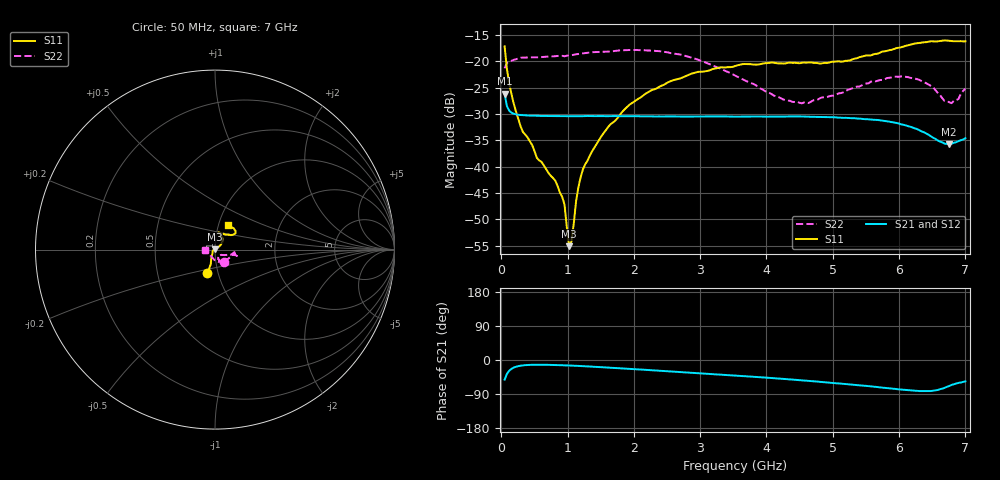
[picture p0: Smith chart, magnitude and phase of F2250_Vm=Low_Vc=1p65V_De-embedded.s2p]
! Integrated Device Technology
! Corporate Headquarters
! 6024 Silver Creek Valley Road
! San Jose, CA 95138  USA
! Phone:  1-408-284-8200
! Toll Free:  1-800-223-1366
! Webpage:  http://www.idt.com/
! Timing and RF Division
! 515 Groton Road, Suite 102
! Westford, MA 01886-6024
! Device:  F2250
! Description: Voltage Variable RF Attenuator
! Frequency:  50.0 -  6000.00 MHz
! Package:  3x3 mm Thin QFN Plastic Package: 16 pin
! Ports:  2 RF, 3 DC
!  Pin  1  = GND
!  Pin  2  = NC
!  Pin  3  = RF1  = Port 1
!  Pin  4  = NC
!  Pin  5  = GND
!  Pin  6  = GND
!  Pin  7  = GND
!  Pin  8  = GND
!  Pin  9  = NC
!  Pin 10  = RF2  = Port 2
!  Pin 11  = NC
!  Pin 12  = GND
!  Pin 13  = GND
!  Pin 14  = VCNTRL
!  Pin 15  = VDD
!  Pin 16  = VMODE
! Vcntrl:  1.650 Volts
! Vmode:  +0.000 Volts
! Vdd:  +3.30  Volts
! Current:  1.189 mA
! Data:  The device was measured on a the F2250 evaluation board which has
!  individual transmission lines to the RF pins.  Data was collected
!  using a calibrated network analyzer.  The evaluation board was
!  de-embedded using a TRL calibration technique.
!  The reference plane is the edge of the package pin.
! Misc:  SN 10
!  Action Tracker AT0258
! Date Measured:  2014-11-26
! Date:  2015-10-15  MJV
! Note:
!  Integrated Device Technology supplies this data as a sample of measured
!  data at the package pin for this product.  Your particular data for this
!  product may vary.
!  Data was taken at 25 degrees C.
!  Integrated Device Technology reserves the right to change this data at anytime.
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# GHz S dB R 50
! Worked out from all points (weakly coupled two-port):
!   201 points, 50 MHz to 7 GHz, reference 50 ohm
!   highest |S21| = -26.13 dB at 50 MHz (marker M1); lowest = -35.7 dB at 6.757 GHz (marker M2)
!   lowest |S11| = -55.1 dB at 1.023 GHz (marker M3), VSWR 1.00, Z = 49.9 + j0.13 ohm
!   |S11| at or under -10 dB: start of sweep to end of sweep
!   |S22| runs from -28.0 to -17.8 dB; largest |S21 - S12| = 0.00018
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0.05  -17.15 -107.7  -26.13 -52.0  -26.10 -51.9  -21.33 -53.1
0.1195  -24.21 -110.2  -29.37 -28.3  -29.39 -28.3  -20.05 -15.7
0.29325  -32.43 -124.5  -30.20 -15.0  -30.19 -15.0  -19.31 -9.0
0.5365  -38.34 -151.2  -30.36 -12.5  -30.38 -12.5  -19.25 -8.3
0.8145  -42.67 174.7  -30.40 -13.2  -30.40 -13.3  -19.02 -11.3
0.91875  -45.75 157.2  -30.41 -13.9  -30.42 -13.9  -18.95 -12.8
0.9535  -47.21 172.4  -30.44 -14.1  -30.42 -14.1  -19.03 -12.9
1.023  -55.12 132.1  -30.43 -14.5  -30.43 -14.5  -18.86 -12.9
1.05775  -54.20 95.7  -30.43 -14.7  -30.43 -14.7  -18.82 -13.0
1.12725  -46.65 47.9  -30.42 -15.3  -30.40 -15.3  -18.65 -14.0
1.2315  -40.51 35.9  -30.42 -16.2  -30.39 -16.2  -18.46 -15.2
1.6485  -31.94 38.8  -30.41 -20.3  -30.40 -20.3  -18.13 -16.0
1.9265  -28.32 39.3  -30.43 -23.3  -30.40 -23.3  -17.85 -16.4
2.37825  -24.87 46.0  -30.47 -28.1  -30.45 -28.1  -18.05 -16.2
3.525  -20.90 71.8  -30.51 -40.9  -30.51 -41.0  -22.70 -24.3
4.25475  -20.42 77.5  -30.49 -49.7  -30.50 -49.7  -27.26 -44.5
4.7065  -20.28 72.0  -30.54 -56.1  -30.52 -56.1  -27.40 -62.8
5.85325  -17.88 40.0  -31.46 -74.8  -31.47 -74.8  -23.13 -71.0
6.305  -16.51 40.3  -33.08 -82.0  -33.09 -82.0  -23.52 -79.7
6.75675  -16.10 50.8  -35.71 -68.5  -35.69 -68.5  -27.77 -133.7
6.89575  -16.15 56.8  -35.16 -60.3  -35.12 -60.4  -27.15 -163.5
7  -16.19 62.9  -34.60 -56.4  -34.58 -56.4  -25.19 -179.5
